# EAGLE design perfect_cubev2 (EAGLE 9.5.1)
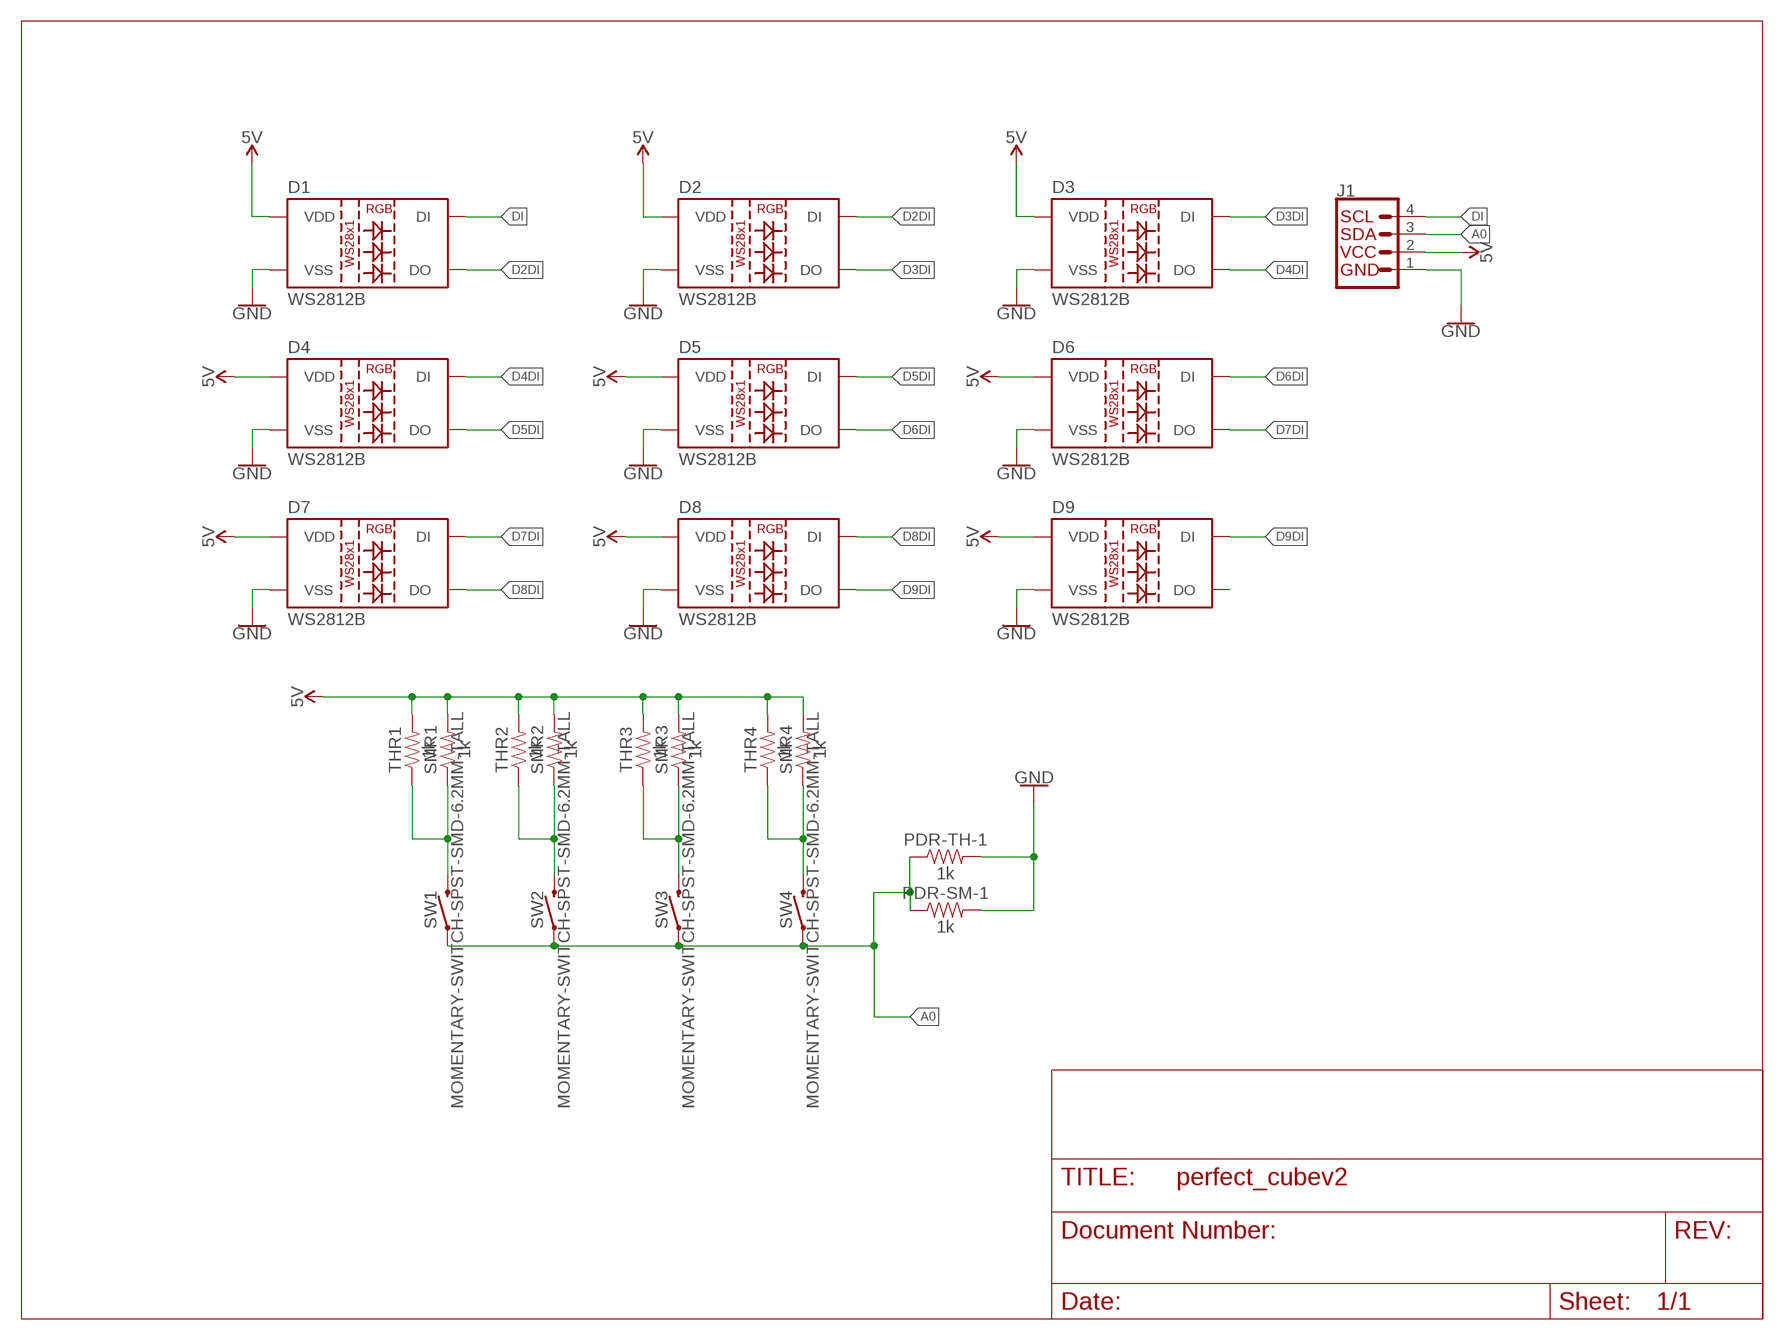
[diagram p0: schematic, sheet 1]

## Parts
D1  WS2812B  [WS2812B]
D2  WS2812B  [WS2812B]
D3  WS2812B  [WS2812B]
D4  WS2812B  [WS2812B]
D5  WS2812B  [WS2812B]
D6  WS2812B  [WS2812B]
D7  WS2812B  [WS2812B]
D8  WS2812B  [WS2812B]
D9  WS2812B  [WS2812B]
J1  QWIIC_CONNECTORJS-1MM  [1X04_1MM_RA]
PDR-SM-1  1k  1KOHM-0603-1/10W-1%  [0603]
PDR-TH-1  1k  1KOHM-HORIZ-1/4W-1%  [AXIAL-0.3]
SMR1  1k  1KOHM-0603-1/10W-1%  [0603]
SMR2  1k  1KOHM-0603-1/10W-1%  [0603]
SMR3  1k  1KOHM-0603-1/10W-1%  [0603]
SMR4  1k  1KOHM-0603-1/10W-1%  [0603]
SW1  MOMENTARY-SWITCH-SPST-SMD-6.2MM-TALL  [TACTILE_SWITCH_SMD_6.2MM_TALL]
SW2  MOMENTARY-SWITCH-SPST-SMD-6.2MM-TALL  [TACTILE_SWITCH_SMD_6.2MM_TALL]
SW3  MOMENTARY-SWITCH-SPST-SMD-6.2MM-TALL  [TACTILE_SWITCH_SMD_6.2MM_TALL]
SW4  MOMENTARY-SWITCH-SPST-SMD-6.2MM-TALL  [TACTILE_SWITCH_SMD_6.2MM_TALL]
THR1  1k  1KOHM-HORIZ-1/4W-1%  [AXIAL-0.3]
THR2  1k  1KOHM-HORIZ-1/4W-1%  [AXIAL-0.3]
THR3  1k  1KOHM-HORIZ-1/4W-1%  [AXIAL-0.3]
THR4  1k  1KOHM-HORIZ-1/4W-1%  [AXIAL-0.3]

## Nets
5V: D1.1(VDD) D2.1(VDD) D3.1(VDD) D4.1(VDD) D5.1(VDD) D6.1(VDD) D7.1(VDD) D8.1(VDD) D9.1(VDD) J1.2(VCC) SMR1.2 SMR2.2 SMR3.2 SMR4.2 THR1.P$2 THR2.P$2 THR3.P$2 THR4.P$2
A0: J1.3(SDA) PDR-SM-1.1 PDR-TH-1.P$1 SW1.A2 SW2.A2 SW3.A2 SW4.A2
D2DI: D1.2(DO) D2.4(DI)
D3DI: D2.2(DO) D3.4(DI)
D4DI: D3.2(DO) D4.4(DI)
D5DI: D4.2(DO) D5.4(DI)
D6DI: D5.2(DO) D6.4(DI)
D7DI: D6.2(DO) D7.4(DI)
D8DI: D7.2(DO) D8.4(DI)
D9DI: D8.2(DO) D9.4(DI)
DI: D1.4(DI) J1.4(SCL)
GND: D1.3(VSS) D2.3(VSS) D3.3(VSS) D4.3(VSS) D5.3(VSS) D6.3(VSS) D7.3(VSS) D8.3(VSS) D9.3(VSS) J1.1(GND) PDR-SM-1.2 PDR-TH-1.P$2
N$1: SMR1.1 SW1.B2 THR1.P$1
N$3: SMR2.1 SW2.B2 THR2.P$1
N$4: SMR3.1 SW3.B2 THR3.P$1
N$5: SMR4.1 SW4.B2 THR4.P$1
Unconnected: D9.2(DO)

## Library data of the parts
D1-D9 = SparkFun-LED:WS2812B: WS2812B SMD addressable RGB LED 5x5mm SMD LED with built-in controller IC. Color: Red/Green/Blue mC Rating: RGB: 390, 660, 180 mcd Forward Voltage: RGB: 2.0, 3.0, 3.0 V Packages:WS2812B SparkFun Products: Blynk Board - ESP8266; PROD_ID: DIO-12503
J1 = SparkFun-Connectors:QWIIC_CONNECTOR: SparkFun I2C Standard Qwiic Connector An SMD 1mm pitch JST connector makes it easy and quick (get it? Qwiic?) to connect I2C devices to each other. The Qwiic system enables fast and solderless connection between popular platforms and various sensors and actuators. We carry 200mm, 100mm, 50mm, and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
PDR-SM-1 SMR1-SMR4 = SparkFun-Resistors:1KOHM: 1kΩ resistor; PROD_ID: RES-07856
PDR-TH-1 THR1-THR4 = SparkFun-Resistors:1KOHM: 1kΩ resistor; PROD_ID: RES-12182
SW1-SW4 = SparkFun-Switches:MOMENTARY-SWITCH-SPST: Momentary Switch (Pushbutton) - SPST; PROD_ID: SWCH-11966; SF_SKU: COM-12992

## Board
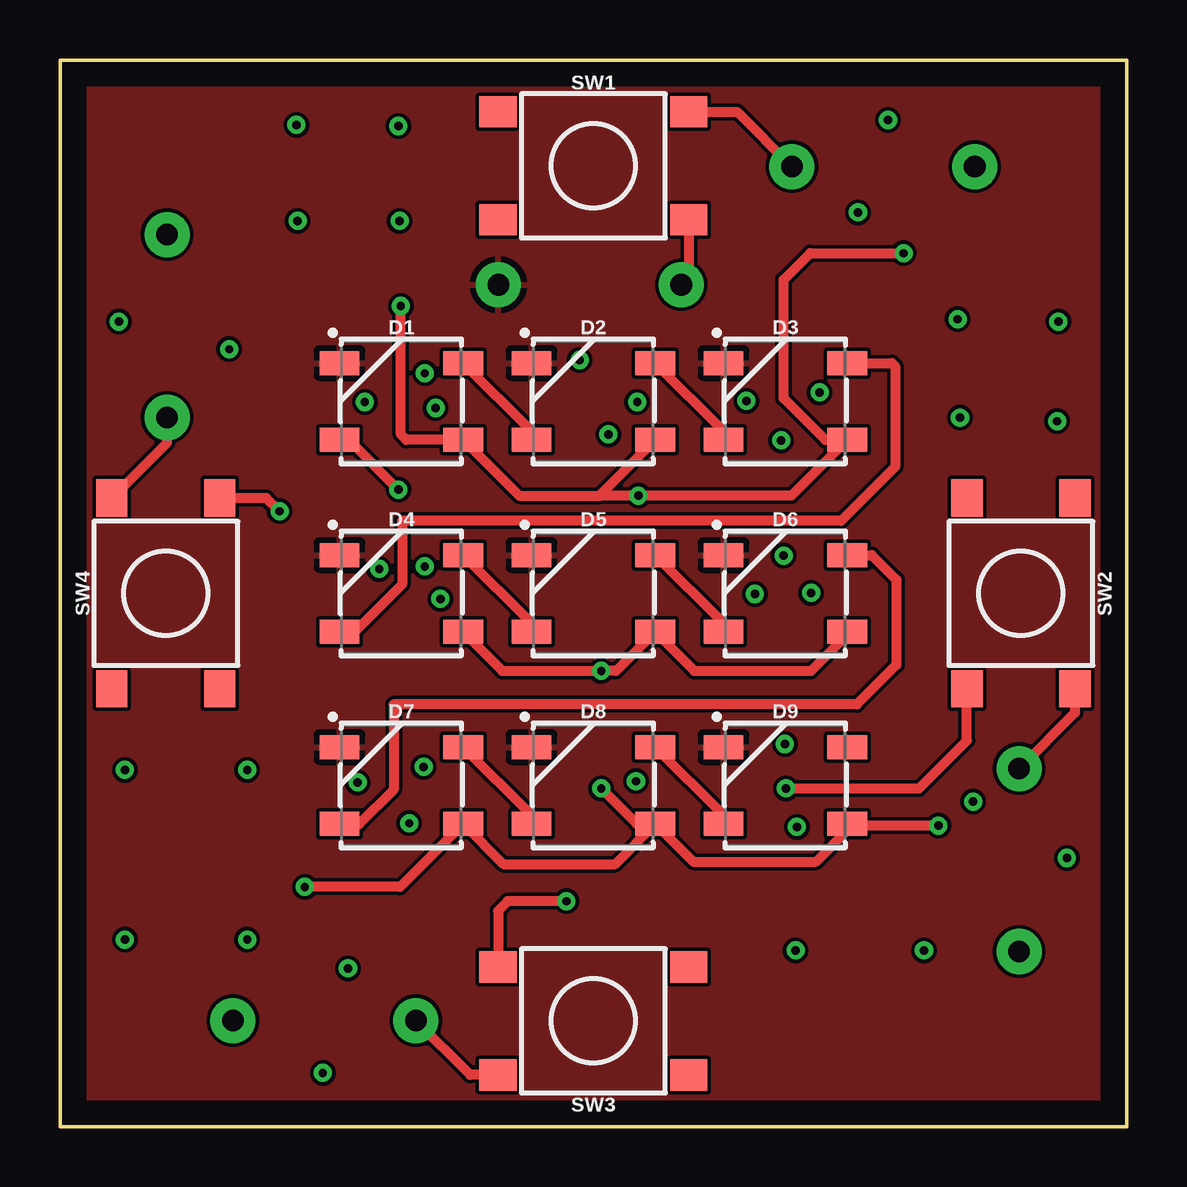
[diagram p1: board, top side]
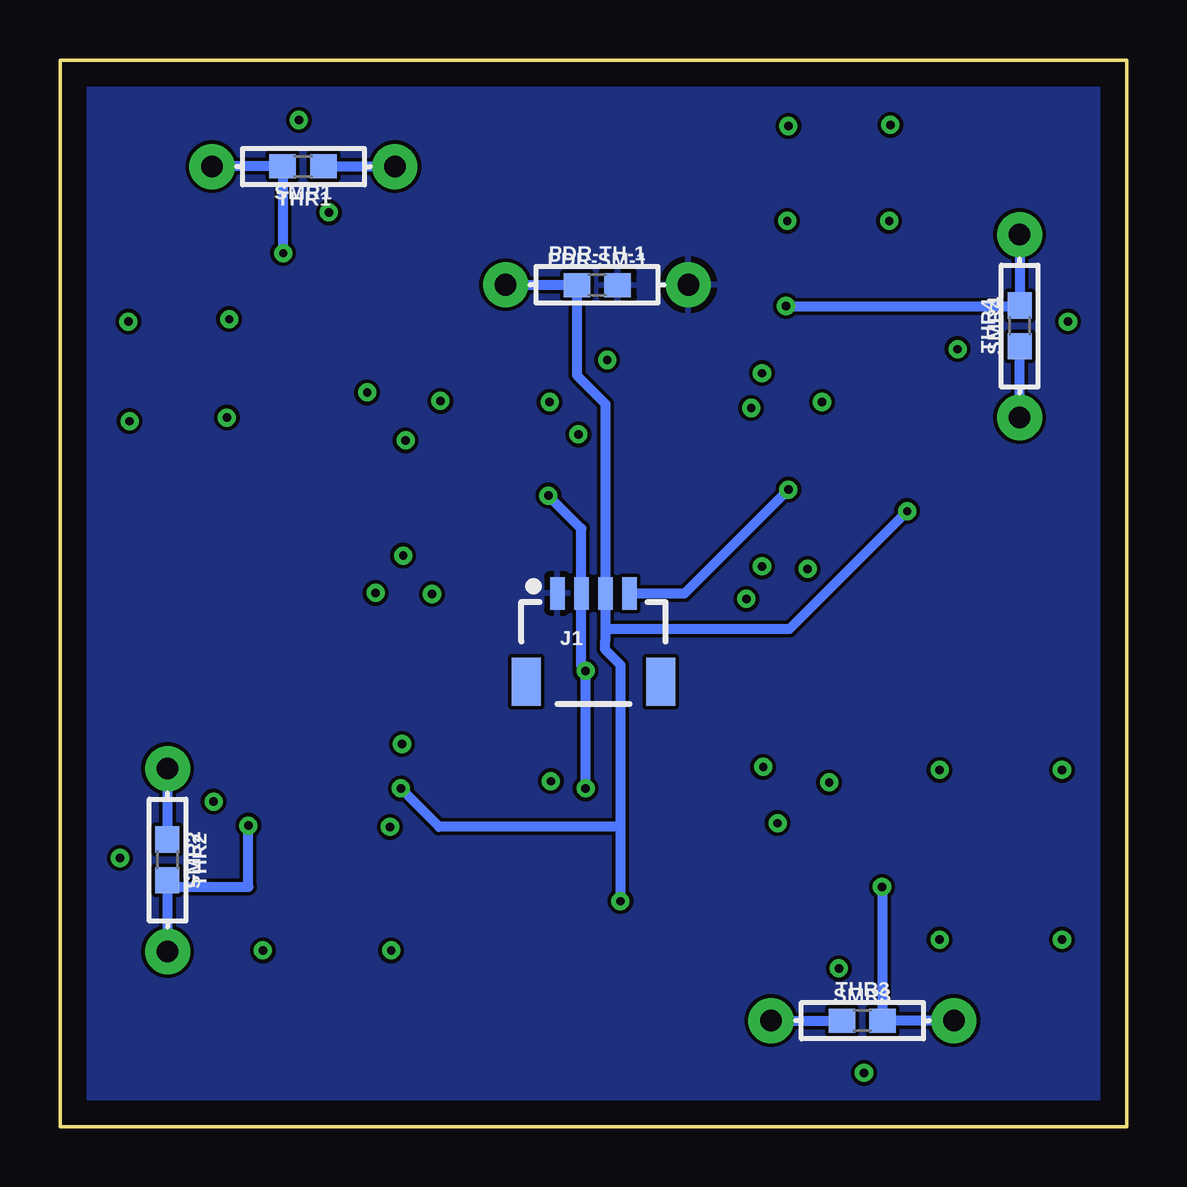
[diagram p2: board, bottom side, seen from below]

Size 44.45 x 44.45 mm. Coordinates in mm from the lower left corner, seen from the top.
Outline: 0,0 0,44.45 44.45,44.45 44.45,0 0,0
Copper layers (1*16): Top 0.035mm / dielectric 1.5mm / Bottom 0.035mm
Design rules "default": minimum track width 6mil, minimum drill 0.35mm, track to track 6mil, track to pad 6mil, pad to pad 6mil, via to via 6mil, smd to smd 6mil, copper to edge 40mil, drill to drill 6mil, minimum pad ring 10mil, minimum via ring 8mil, stop-mask expansion 4mil, vias tented up to drill 0mil, thermal gap 10mil

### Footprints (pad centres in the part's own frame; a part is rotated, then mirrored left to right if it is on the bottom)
WS2812B = smd 1.651 x 1: 1 2.577,-1.6; 2 2.577,1.6; 3 -2.577,1.6; 4 -2.577,-1.6
1X04_1MM_RA = smd 0.6 x 1.35: 1 -1.5,0; 2 -0.5,0; 3 0.5,0; 4 1.5,0 | smd 1.2 x 2: NC1 2.8,-3.675; NC2 -2.8,-3.675
0603 = smd 1.1 x 1: 1 -0.85,0; 2 0.85,0
AXIAL-0.3 = drill 0.9 pad 1.88: P$1 -3.81,0; P$2 3.81,0
TACTILE_SWITCH_SMD_6.2MM_TALL = smd 1.55 x 1.3: A1 -3.975,-2.25; A2 3.975,-2.25; B1 -3.975,2.25; B2 3.975,2.25

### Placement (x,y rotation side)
D1  14.22,30.23 0 top
D2  22.23,30.23 0 top
D3  30.23,30.23 0 top
D4  14.22,22.23 0 top
D5  22.23,22.23 0 top
D6  30.23,22.23 0 top
D7  14.22,14.22 0 top
D8  22.23,14.22 0 top
D9  30.23,14.22 0 top
J1  22.23,22.23 0 bottom
PDR-SM-1  22.07,35.06 0 bottom
PDR-TH-1  22.07,35.09 0 bottom
SMR1  34.33,40.02 180 bottom
SMR2  39.98,11.12 270 bottom
SMR3  11.03,4.42 0 bottom
SMR4  4.46,33.38 90 bottom
SW1  22.23,40.04 0 top
SW2  40.04,22.23 270 top
SW3  22.23,4.41 180 top
SW4  4.41,22.23 90 top
THR1  34.3,40.01 180 bottom
THR2  39.97,11.12 270 bottom
THR3  11.02,4.42 0 bottom
THR4  4.46,33.37 90 bottom

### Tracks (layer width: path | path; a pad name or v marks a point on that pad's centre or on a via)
5V  (via drill 0.35)
  Top 0.406: THR3.P$2 7.1,4.53 | 32.83,20.6 D6.1 32.8,20.5 31.3,19 26.43,19 D5.1 23.18,19 v22.55,19 18.43,19 D4.1 | 22.55,26.3 19.13,26.3 D1.1 14.43,28.62 14.2,28.85 v14.2,34.2 | D2.1 22.55,26.37 22.55,26.3 | 22.55,26.3 v24.1,26.3 30.48,26.3 D3.1 31.88,28.62 30.15,30.35 30.15,35.3 31.25,36.4 v35.15,36.4 | D8.1 23.13,10.95 18.48,10.95 D7.1 14.18,10 v10.2,10 | D8.1 26.38,11.05 31.5,11.05 32.8,12.35 D9.1 32.88,12.55 v36.6,12.55 | D8.1 24.02,12.62 v22.55,14.1
  Bottom 0.406: THR4.P$2 SMR4.2 | SMR4.2 | THR1.P$2 38.1,40.02 SMR1.2 35.15,39.99 v35.15,36.4 | THR2.P$2 39.97,10.27 SMR2.2 39.7,10 36.6,10 v36.6,12.55 | THR3.P$2 10.16,4.42 | 10.16,4.42 SMR3.2 | v22.55,14.1 v22.55,19 22.73,19.18 J1.2 22.73,24.93 v24.1,26.3 | v14.2,34.2 4.5,34.2 SMR4.2 | v10.2,10 10.2,4.46 10.16,4.42
A0  (via drill 0.35)
  Top 0.406: SW1.A2 26.2,35.4 PDR-TH-1.P$1 | 37.69,18.15 SW2.A2 37.79,16.09 35.8,14.1 v30.25,14.1 | v21.1,9.4 18.65,9.4 18.25,9 SW3.A2 | v9.15,25.65 8.6,26.2 SW4.A2
  Bottom 0.406: PDR-TH-1.P$1 22.93,35.09 PDR-SM-1.1 22.91,31.32 21.73,30.12 J1.3 21.73,20.6 | 21.73,20.6 21.73,20.27 21.75,20.25 21.75,19.9 21.1,19.25 21.1,12.5 | 21.1,12.5 v21.1,9.4 | 21.73,20.6 21.57,20.75 14.05,20.75 v9.15,25.65 | 21.1,12.5 28.65,12.5 v30.25,14.1
D2DI
  Top 0.406: D1.2 19.65,28.98 D2.4
D3DI
  Top 0.406: D2.2 27.65,28.98 D3.4
D4DI
  Top 0.406: D3.2 34.67,31.82 34.8,31.7 34.8,27.5 32.55,25.25 14.25,25.25 14.25,22.6 12.28,20.62 D4.4
D5DI
  Top 0.406: D4.2 19.65,20.98 D5.4
D6DI
  Top 0.406: D5.2 27.65,20.98 D6.4
D7DI
  Top 0.406: D6.2 33.83,23.82 34.85,22.8 34.85,19.25 33.2,17.6 13.9,17.6 13.9,14.05 12.47,12.62 D7.4
D8DI
  Top 0.406: D7.2 19.65,12.98 D8.4
D9DI
  Top 0.406: D8.2 27.65,12.98 D9.4
DI  (via drill 0.35)
  Top 0.406: v14.1,26.55 12.03,28.62 D1.4
  Bottom 0.406: J1.4 18.43,22.23 v14.1,26.55
GND
  pour Top: 0,44 44,44 44,0 0,0
  pour Bottom: 0,44 44,44 44,0 0,0
N$1
  Top 0.406: SW1.B2 28.21,42.29 THR1.P$1
  Bottom 0.406: THR1.P$1 33.47,40.01 SMR1.1
N$2  (via drill 0.35)
  other vias: 2.7,7.8
N$3
  Top 0.406: SW2.B2 42.29,17.25 THR2.P$1
  Bottom 0.406: THR2.P$1 39.98,14.91 SMR2.1
N$4
  Top 0.406: SW3.B2 17.09,2.16 THR3.P$1
  Bottom 0.406: THR3.P$1 SMR3.1
N$5
  Top 0.406: SW4.B2 4.46,28.5 THR4.P$1
  Bottom 0.406: THR4.P$1 SMR4.1
N$6  (via drill 0.35)
  other vias: 7.8,7.8
N$7  (via drill 0.35)
  other vias: 2.7,14.88
N$8  (via drill 0.35)
  other vias: 7.8,14.88
N$9  (via drill 0.35)
  other vias: 30.65,7.35
N$10  (via drill 0.35)
  other vias: 36,7.35
N$11  (via drill 0.35)
  other vias: 37.5,29.55
N$12  (via drill 0.35)
  other vias: 37.4,33.65
N$13  (via drill 0.35)
  other vias: 41.6,33.55
N$14  (via drill 0.35)
  other vias: 41.55,29.4
N$15  (via drill 0.35)
  other vias: 14.15,37.75
N$16  (via drill 0.35)
  other vias: 9.9,37.75
N$17  (via drill 0.35)
  other vias: 9.85,41.75
N$18  (via drill 0.35)
  other vias: 14.1,41.7
N$19  (via drill 0.35)
  other vias: 24.05,30.2
N$20  (via drill 0.35)
  other vias: 22.85,28.85
N$21  (via drill 0.35)
  other vias: 21.65,31.95
N$22  (via drill 0.35)
  other vias: 30.05,28.6
N$23  (via drill 0.35)
  other vias: 28.6,30.25
N$24  (via drill 0.35)
  other vias: 31.65,30.6
N$25  (via drill 0.35)
  other vias: 12.7,30.2
N$26  (via drill 0.35)
  other vias: 15.65,29.95
N$27  (via drill 0.35)
  other vias: 15.2,31.4
N$28  (via drill 0.35)
  other vias: 15.2,23.35
N$29  (via drill 0.35)
  other vias: 15.85,22
N$30  (via drill 0.35)
  other vias: 13.3,23.25
N$31  (via drill 0.35)
  other vias: 30.15,23.8
N$32  (via drill 0.35)
  other vias: 28.95,22.2
N$33  (via drill 0.35)
  other vias: 31.3,22.25
N$34  (via drill 0.35)
  other vias: 30.2,15.95
N$35  (via drill 0.35)
  other vias: 30.7,12.5
N$36  (via drill 0.35)
  other vias: 24,14.4
N$37  (via drill 0.35)
  other vias: 15.15,15
N$38  (via drill 0.35)
  other vias: 14.55,12.65
N$39  (via drill 0.35)
  other vias: 12.4,14.35
N$40  (via drill 0.35)
  other vias: 7.05,32.4
N$41  (via drill 0.35)
  other vias: 33.25,38.1
N$42  (via drill 0.35)
  other vias: 41.95,11.2
N$43  (via drill 0.35)
  other vias: 12,6.6
N$44  (via drill 0.35)
  other vias: 2.45,33.55
N$45  (via drill 0.35)
  other vias: 34.5,41.95
N$46  (via drill 0.35)
  other vias: 10.95,2.25
N$47  (via drill 0.35)
  other vias: 38.05,13.55

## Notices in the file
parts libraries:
SparkFun-LED: Licensing: Creative Commons ShareAlike 4.0 International - https://creativecommons.org/licenses/by-sa/4.0
